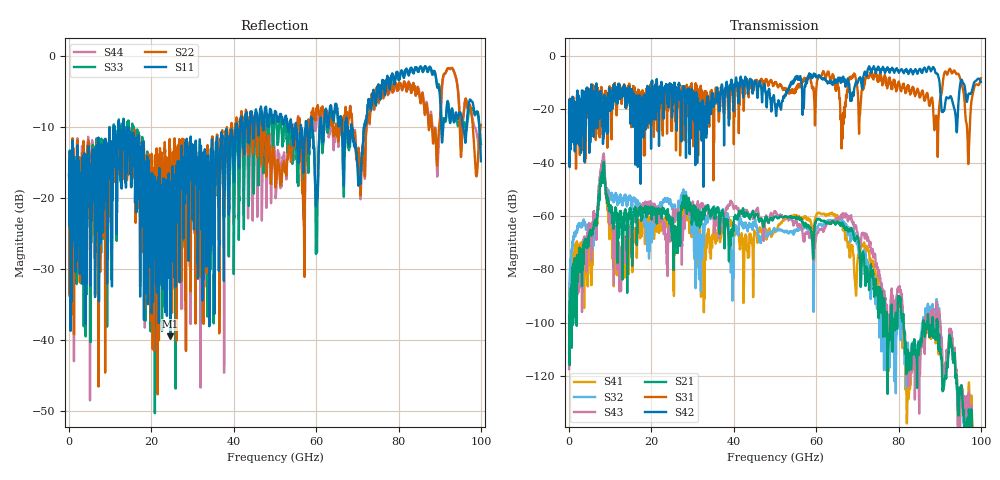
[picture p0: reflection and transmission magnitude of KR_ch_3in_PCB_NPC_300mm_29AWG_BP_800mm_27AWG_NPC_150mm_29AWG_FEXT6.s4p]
# GHz S RI R 45
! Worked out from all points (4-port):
!   4000 points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, 25 MHz to 100 GHz, reference 45 ohm
!   strongest paths, dB at 25 MHz, 25.02 GHz, 50.02 GHz, 75.03 GHz, 100 GHz:
!     S42: -21.2, -20.7, -18.6, -4.1, -9.8
!     S31: -21.3, -21.0, -10.2, -8.8, -8.4
!     S21: -108.4, -67.8, -60.2, -89.4, -160.4
!     S43: -117.3, -61.5, -58.1, -81.1, -153.5
!     S32: -98.4, -57.0, -65.1, -91.6, -178.6
!     S41: -105.0, -67.2, -65.9, -84.6, -154.3
!   lowest |S11| = -39.4 dB at 24.62 GHz (marker M1), VSWR 1.02, Z = 44.1 + j0.388 ohm
!   |S11| at or under -10 dB: start of sweep to 10.87 GHz; 14.28 GHz to 40.62 GHz (26.34 GHz wide, 96 % of centre); 68.66 GHz to 71.57 GHz (2.915 GHz wide, 4.16 % of centre)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
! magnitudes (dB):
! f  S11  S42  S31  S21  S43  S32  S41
! 25 MHz  -16.8  -21.2  -21.3  -108.4  -117.3  -98.4  -105.0
! 8.1 GHz  -15.3  -19.4  -16.6  -46.8  -41.8  -45.0  -43.3
! 12.38 GHz  -11.6  -16.1  -12.7  -58.1  -78.2  -52.0  -77.6
! 24.62 GHz  -39.4  -13.2  -15.8  -61.4  -63.3  -54.2  -61.6
! 92.5 GHz  -9.4  -15.2  -4.9  -105.0  -102.3  -103.8  -103.3
! 96.88 GHz  -7.5  -15.0  -38.3  -137.7  -133.2  -142.4  -129.2
! 100 GHz  -14.8  -9.8  -8.4  -160.4  -153.5  -178.6  -154.3
